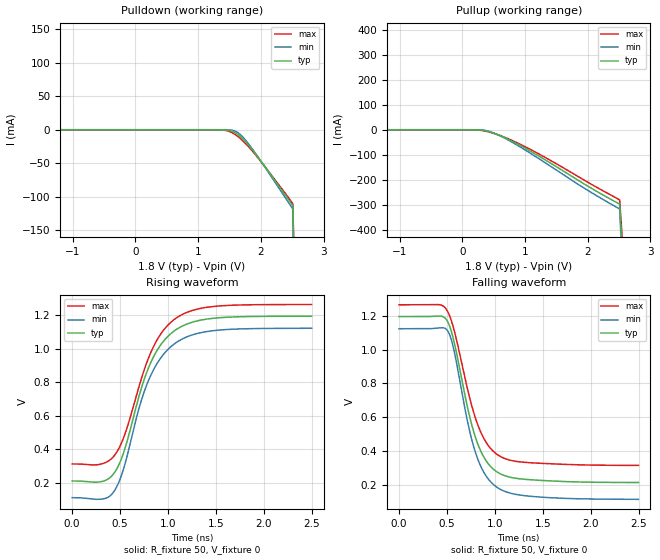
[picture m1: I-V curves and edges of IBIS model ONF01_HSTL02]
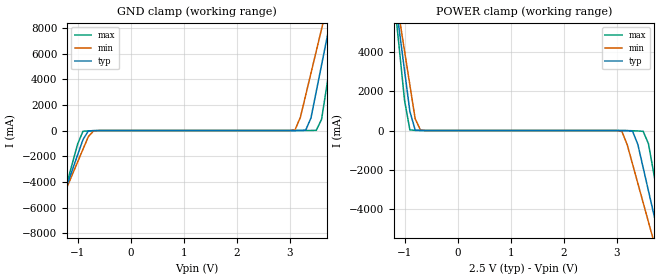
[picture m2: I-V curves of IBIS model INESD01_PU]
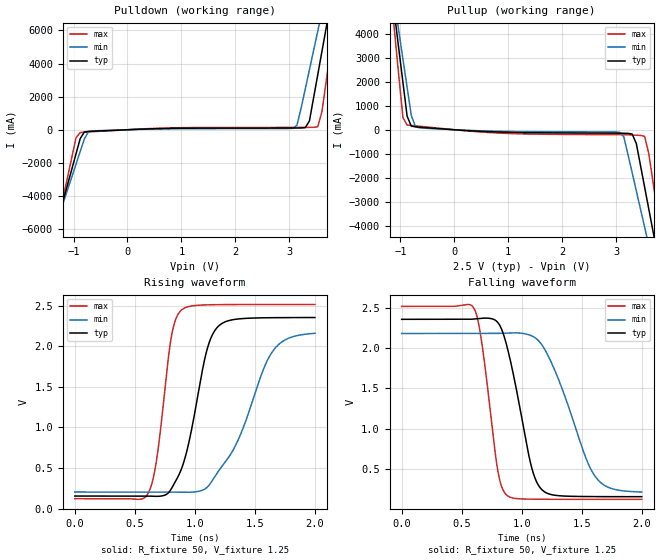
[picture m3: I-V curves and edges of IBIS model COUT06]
|   This file is an IBIS representation of the   |
|   Integrated Device Technology , Inc.   |
|   ICS8427-02   |
|   500MHZ, LOW JITTER LVCMOS/CRYSTALTO-LVHSTL FREQUENCY SYNTHESIZER   |
[IBIS Ver]   4.1
[File name]   8427_02_2v5.ibs
[File Rev]   1.0
[Date]   2 Sep 2009 | Last modified
|   Sep 29 2004 | Generated
[Source]   Originated at Integrated Device Technology, Inc.
[Disclaimer]
IDT hereby grants the user of this IBIS model a non-exclusive,
nontransferable license to use this IBIS model under the following terms.
Before using this IBIS model, the user should read this license.
If the user does not accept these terms,  the IBIS model should be
returned to IDT within 30 days.
   The user is granted this license only to use the IBIS model and
is not granted rights to sell, load, rent, lease or license the IBIS
model in whole or in part, or in modified form to anyone other than
user. User may modify the IBIS model to suit its specific
applications but rights to derivative works and such modifications
shall belong to IDT.
   This IBIS model is provided on an "AS IS" basis and IDT makes
absolutely no warranty with respect to the information contained
herein. IDT DISCLAIMS AND CUSTOMER WAIVES ALL WARRANTIES, EXPRESS
OR IMPLIED, INCLUDING WARRANTIES OF MERCHANTABILITY OR FITNESS FOR
A PARTICULAR PURPOSE. The entire risk as to quality and performance
is with the Customer. ACCORDINGLY, IN NO EVENT SHALL THE COMPANY BE
LIABLE FOR ANY DAMAGES, WHETHER IN CONTRACT OR TORT,INCLUDING ANY
LOST PROFITS OR OTHER INCIDENTAL, CONSEQUENTIAL, EXEMPLARY, OR
PUNITIVE DAMAGES ARISING OUT OF THE USE OR APPLICATION OF THE IBIS
model provided in this package. Further, IDT reserves the right to
make changes without notice to any product herein to improve
reliability, function, or design. IDT does not convey any license
under patent rights or any other intellectual property rights,
including those of third parties.
   IDT is not obligated to provide maintenance or support
for the licensed IBIS model.
[Copyright]   Copyright 2004 by Integrated Device Technology , Inc.
[Component]   ICS8427Y-02
[Manufacturer] Integrated Device Technology, Inc.
[Package]
|LQFP32
|lead + wire   typ   min   max
R_pkg   220.4m   212.5m   238m
L_pkg   1.841n   1.708n   1.974n
C_pkg   0.316p   0.2907p   0.33p
[Pin]   signal_name   model_name   R_pin   L_pin   C_pin
1   VDDO   POWER   238m   1.974n   0.330p
2   FOUT2   ONF01_HSTL02   225m   1.841n   0.311p
3   nFOUT2   ONF01_HSTL02   218m   1.7745n   0.301p
4   VDDO   POWER   213m   1.708n   0.291p
5   FOUT3   ONF01_HSTL02   213m   1.708n   0.291p
6   nFOUT3   ONF01_HSTL02   218m   1.7745n   0.301p
7   OE   INESD01_PU   225m   1.841n   0.311p
8   GND   GND   238m   1.974n   0.330p
9   TEST   COUT06   238m   1.974n   0.330p
10   VDD   POWER   225m   1.841n   0.311p
11   FOUT4   ONF01_HSTL02   218m   1.7745n   0.301p
12   nFOUT4   ONF01_HSTL02   213m   1.708n   0.291p
13   VDDO   POWER   213m   1.708n   0.291p
14   FOUT5   ONF01_HSTL02   218m   1.7745n   0.301p
15   nFOUT5   ONF01_HSTL02   225m   1.841n   0.311p
16   GND   GND   238m   1.974n   0.330p
17   MR   INESD01_PD   238m   1.974n   0.330p
18   S_CLOCK   INESD01_PD   225m   1.841n   0.311p
19   S_DATA   INESD01_PD   218m   1.7745n   0.301p
20   S_LOAD   INESD01_PD   213m   1.708n   0.291p
21   VDDA   POWER   213m   1.708n   0.291p
22   XTAL_SEL   INESD01_PU   218m   1.7745n   0.301p
23   TEST_CLK   INESD01_PD   225m   1.841n   0.311p
24   XTAL_OUT   NC   238m   1.974n   0.330p
25   XTAL_IN   NC   238m   1.974n   0.330p
26   VDD   POWER   225m   1.841n   0.311p
27   VCO_SEL   INESD01_PU   218m   1.7745n   0.301p
28   FOUT0   ONF01_HSTL02   213m   1.708n   0.291p
29   nFOUT0   ONF01_HSTL02   213m   1.708n   0.291p
30   VDDO   POWER   218m   1.7745n   0.301p
31   FOUT1   ONF01_HSTL02   225m   1.841n   0.311p
32   nFOUT1   ONF01_HSTL02   238m   1.974n   0.330p
[Diff Pin]  inv_pin  vdiff tdelay_typ tdelay_min  tdelay_max
2   3   NA   0   0   0
5   6   NA   0   0   0
11   12   NA   0   0   0
14   15   NA   0   0   0
28   29   NA   0   0   0
31   32   NA   0   0   0
[Component]   ICS8427K-02
[Manufacturer] Integrated Device Technology, Inc.
[Package]
|LD QFN 32
|lead + wire   typ   min   max
R_pkg   72.4655m   58.886m   86.045m
L_pkg   1.47175nH   1.11650nH   1.77850nH
C_pkg   0.07747pF   0.07444pF   0.08050pF
[Pin]   signal_name   model_name   R_pin   L_pin   C_pin
1   VDDO   POWER   86.045m   1.77850nH   0.08050pF
2   FOUT2   ONF01_HSTL02   76.996m   1.55783nH   0.07848pF
3   nFOUT2   ONF01_HSTL02   67.941m   1.33717nH   0.07646pF
4   VDDO   POWER   58.886m   1.11650nH   0.07444pF
5   FOUT3   ONF01_HSTL02   58.886m   1.11650nH   0.07444pF
6   nFOUT3   ONF01_HSTL02   67.941m   1.33717nH   0.07646pF
7   OE   INESD01_PU   76.996m   1.55783nH   0.07848pF
8   GND   GND   86.045m   1.77850nH   0.08050pF
9   TEST   COUT06   86.045m   1.77850nH   0.08050pF
10   VDD   POWER   76.996m   1.55783nH   0.07848pF
11   FOUT4   ONF01_HSTL02   67.941m   1.33717nH   0.07646pF
12   nFOUT4   ONF01_HSTL02   58.886m   1.11650nH   0.07444pF
13   VDDO   POWER   58.886m   1.11650nH   0.07444pF
14   FOUT5   ONF01_HSTL02   67.941m   1.33717nH   0.07646pF
15   nFOUT5   ONF01_HSTL02   76.996m   1.55783nH   0.07848pF
16   GND   GND   86.045m   1.77850nH   0.08050pF
17   MR   INESD01_PD   86.045m   1.77850nH   0.08050pF
18   S_CLOCK   INESD01_PD   76.996m   1.55783nH   0.07848pF
19   S_DATA   INESD01_PD   67.941m   1.33717nH   0.07646pF
20   S_LOAD   INESD01_PD   58.886m   1.11650nH   0.07444pF
21   VDDA   POWER   58.886m   1.11650nH   0.07444pF
22   XTAL_SEL   INESD01_PU   67.941m   1.33717nH   0.07646pF
23   TEST_CLK   INESD01_PD   76.996m   1.55783nH   0.07848pF
24   XTAL_OUT   NC   86.045m   1.77850nH   0.08050pF
25   XTAL_IN   NC   86.045m   1.77850nH   0.08050pF
26   VDD   POWER   76.996m   1.55783nH   0.07848pF
27   VCO_SEL   INESD01_PU   67.941m   1.33717nH   0.07646pF
28   FOUT0   ONF01_HSTL02   58.886m   1.11650nH   0.07444pF
29   nFOUT0   ONF01_HSTL02   58.886m   1.11650nH   0.07444pF
30   VDDO   POWER   67.941m   1.33717nH   0.07646pF
31   FOUT1   ONF01_HSTL02   76.996m   1.55783nH   0.07848pF
32   nFOUT1   ONF01_HSTL02   86.045m   1.77850nH   0.08050pF
[Diff Pin]  inv_pin  vdiff tdelay_typ tdelay_min  tdelay_max
2   3   NA   0   0   0
5   6   NA   0   0   0
11   12   NA   0   0   0
14   15   NA   0   0   0
28   29   NA   0   0   0
31   32   NA   0   0   0
| Models and submodels in the file (4): ONF01_HSTL02 (Output_ECL), INESD01_PU (Input), COUT06 (Output), INESD01_PD (Input)
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[Model]   ONF01_HSTL02
Model_type   Output_ECL
Polarity   Non-Inverting
|   typ   min   max
C_comp   2pF   1.5pF   2.5pF
Vmeas = 0.713V
Rref = 50
Cref = 0
Vref = 0V
|   typ   min   max
[Voltage range]   1.8V   1.71V   1.89V
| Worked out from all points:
|   rising waveform, R_fixture 50, V_fixture 0: 20-80 % time 341ps typ, 342ps min, 349ps max; typ from 0.212 V to 1.2 V
|   falling waveform, R_fixture 50, V_fixture 0: 20-80 % time 252ps typ, 248ps min, 265ps max; typ from 1.2 V to 0.212 V
[Pulldown]
|Voltage   I (typ)   I (min)   I (max)
-2.5V     3.779A     4.549A     3.324A
-1.7V     586.5mA    472mA      663.2mA
-1.5V     6.551mA    1.102mA    39.5mA
-1.49V    4.852mA    904.9uA    29.1mA
-1.444V   1.516mA    377.5uA    7.658mA
-1.352V   257.5uA    51.81uA    872.2uA
1.308V    -7.57uA    -216.9nA   -66.94uA
1.583V    -3.964mA   -1.674mA   -6.635mA
1.858V    -29.26mA   -27.71mA   -30.99mA
2.51V     -113.3mA   -118mA     -110.4mA
3.008V    -2.414A    -3.03A     -2.033A
5V        -14.82A    -18.84A    -12.39A
[Pullup]
|Voltage   I (typ)   I (min)   I (max)
-2.5V     3.779A     4.549A     3.324A
-1.7V     586.5mA    472mA      663.3mA
-1.5V     6.553mA    1.102mA    39.51mA
-1.444V   1.517mA    377.6uA    7.668mA
-1.352V   258.7uA    51.85uA    882uA
161mV     -70.79uA   -10.25uA   -233.3uA
482.1mV   -12.19mA   -11.14mA   -12.94mA
1.124V    -91.36mA   -100.4mA   -83.99mA
1.904V    -211.2mA   -227.8mA   -196mA
2.51V     -298.8mA   -317.6mA   -281.4mA
3.008V    -2.601A    -3.23A     -2.207A
5V        -15.01A    -19.04A    -12.57A
[Ramp]
|   typ   min   max
dV/dt_r   0.792/0.556n   0.816/0.558n   0.765/0.565n
dV/dt_f   0.789/0.399n   0.813/0.398n   0.762/0.417n
R_load =   50.0000
[Rising Waveform]
R_fixture = 50
V_fixture = 0
V_fixture_max = 0
V_fixture_min = 0
C_fixture = 0.0p
| Time   typ   min   max
0s        212mV      112.4mV    313.4mV
300.3ps   207.8mV    103.5mV    312.7mV
437.9ps   259.1mV    150.9mV    362mV
553.1ps   409.3mV    316.6mV    495.2mV
695.7ps   713.5mV    641.9mV    772mV
793.3ps   882.6mV    807.1mV    940.9mV
920.9ps   1.022V     943.4mV    1.086V
1.076ns   1.112V     1.034V     1.18V
1.486ns   1.184V     1.11V      1.254V
2.498ns   1.195V     1.123V     1.265V
[Falling Waveform]
R_fixture = 50
V_fixture = 0
V_fixture_max = 0
V_fixture_min = 0
C_fixture = 0.0p
| Time   typ   min   max
0s        1.195V     1.123V     1.265V
420.4ps   1.199V     1.128V     1.266V
510.5ps   1.162V     1.108V     1.222V
570.6ps   1.055V     1.003V     1.125V
710.7ps   667.1mV    584.1mV    775.4mV
790.8ps   491.1mV    402.1mV    605.3mV
890.9ps   356.7mV    266.7mV    467.3mV
1.016ns   277.2mV    186mV      381.6mV
1.394ns   227.6mV    129.5mV    328.5mV
2.498ns   212.2mV    112.6mV    313.6mV
[Model]   INESD01_PU
Model_type   Input
Polarity   Non-Inverting
Vinl = 1.4V
Vinh = 1.85V
|   typ   min   max
C_comp   2pF   1.5pF   2.5pF
|   typ   min   max
[Voltage range]  2.5V   2.375V   2.625V
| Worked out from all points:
|   GND clamp passes 1 mA (typ) near -0.54 V on its own axis
|   POWER clamp passes 1 mA (typ) near -0.66 V on its own axis
[GND_clamp]
|Voltage   I(typ)   I(min)   I(max)
-2.5V     -19.6A     -17.18A    -23.67A
-1.6V     -8.969A    -8.332A    -10.1A
-1.5V     -7.788A    -7.349A    -8.588A
-900mV    -707.1mA   -1.46A     -57.43mA
-700mV    -7.027mA   -24.05mA   -13.28mA
3.1V      199.2uA    53.94mA    11.78uA
3.3V      28.4mA     2.748A     652.4uA
3.5V      3.045A     6.192A     15.72mA
3.6V      5.115A     7.914A     872.4mA
3.7V      7.185A     9.638A     3.52A
3.9V      11.33A     13.09A     8.818A
5V        34.14A     32.07A     37.99A
[POWER_clamp]
|Voltage   I(typ)   I(min)   I(max)
-1.5V     9.257A     9.207A     9.48A
-1.2V     7.185A     7.484A     6.83A
-1.1V     5.115A     5.761A     4.182A
-900mV    976.9mA    2.318A     34.23mA
-700mV    1.582mA    24.31mA    1.044mA
3.1V      -2.107mA   -51.03mA   -534.5uA
3.3V      -35.62mA   -1.705A    -10.86mA
3.5V      -1.886A    -3.666A    -39.41mA
3.6V      -3.066A    -4.647A    -666.9mA
3.8V      -5.426A    -6.612A    -3.684A
3.9V      -6.607A    -7.595A    -5.193A
5V        -19.6A     -18.41A    -21.79A
[Model]   COUT06
Model_type   Output
Polarity   Non-Inverting
|   typ   min   max
C_comp   2pF   1.5pF   2.5pF
Vmeas = 1.25V
Rref = 50
Vref = 1.25V
|   typ   min   max
[Voltage range]   2.5V   2.375V   2.625V
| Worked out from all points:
|   slope of the pulldown table from 0 to 0.375 V, typ, clamps not added: 7.84 ohm
|   slope of the pullup table from 0 to 0.375 V, typ, clamps not added: 7.16 ohm
|   rising waveform, R_fixture 50, V_fixture 1.25: 20-80 % time 181ps typ, 322ps min, 114ps max; typ from 0.154 V to 2.35 V
|   falling waveform, R_fixture 50, V_fixture 1.25: 20-80 % time 175ps typ, 285ps min, 118ps max; typ from 2.35 V to 0.154 V
[pulldown]
|Voltage   I (typ)   I (min)   I (max)
-2.5V     -19.75A    -17.31A    -23.85A
-1.34V    -6.031A    -5.882A    -6.333A
-953.6mV  -1.449A    -2.071A    -479.4mA
-876.3mV  -533mA     -1.309A    -169.7mA
-644.3mV  -89.97mA   -69.78mA   -117.4mA
3.067V    103.7mA    87.56mA    139.5mA
3.144V    104.2mA    267.1mA    139.8mA
3.376V    532mA      3.625A     142.7mA
3.531V    3.329A     5.955A     178.4mA
3.686V    6.13A      8.286A     2.887A
3.84V     8.933A     10.62A     6.471A
5V        29.99A     28.14A     33.4A
[pullup]
|Voltage   I (typ)   I (min)   I (max)
-2.5V     30.11A     26.36A     36.43A
-1.108V   4.788A     5.285A     4.064A
-1.031V   3.38A      4.114A     2.264A
-953.6mV  1.972A     2.943A     504.8mA
-876.3mV  566.5mA    1.772A     199.4mA
-799mV    152.8mA    600.7mA    177mA
3.067V    -143.2mA   -109.6mA   -206.5mA
3.299V    -177.9mA   -1.786A    -218.7mA
3.531V    -2.395A    -4.061A    -274.9mA
3.686V    -4.221A    -5.58A     -2.168A
3.84V     -6.047A    -7.1A      -4.502A
5V        -19.75A    -18.51A    -22.01A
[Ramp]
|   typ   min   max
dV/dt_r   1.50/0.6n   1.50/0.80n   1.50/0.4n
dV/dt_f   1.50/0.6n   1.50/0.80n   1.50/0.4n
[Rising Waveform]
R_fixture = 50
V_fixture = 1.25
V_fixture_max = 1.3125
V_fixture_min = 1.1875
C_fixture = 0.0p
0s        154.1mV    203.2mV    121.3mV
609ps     154.1mV    203.2mV    184mV
682.5ps   150.3mV    203.3mV    612.2mV
806.4ps   249.2mV    203.4mV    2.136V
892.5ps   505.9mV    202.2mV    2.452V
1.094ns   1.919V     251.9mV    2.51V
1.184ns   2.23V      435mV      2.513V
1.359ns   2.337V     840.1mV    2.515V
1.646ns   2.353V     1.935V     2.515V
1.999ns   2.355V     2.16V      2.515V
[Falling Waveform]
R_fixture = 50
V_fixture = 1.25
V_fixture_max = 1.3125
V_fixture_min = 1.1875
C_fixture = 0.0p
0s        2.355V     2.179V     2.515V
602.7ps   2.358V     2.179V     2.489V
665.7ps   2.367V     2.179V     2.08V
802.2ps   2.313V     2.18V      463.4mV
877.8ps   2.013V     2.185V     169.6mV
1.073ns   571.7mV    2.155V     123.2mV
1.161ns   250.7mV    2.051V     122mV
1.296ns   167.9mV    1.648V     121.4mV
1.606ns   155.1mV    416.2mV    121.3mV
1.999ns   154.1mV    211.8mV    121.3mV
